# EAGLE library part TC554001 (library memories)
Static RAM 512K x 8 bits Toshiba
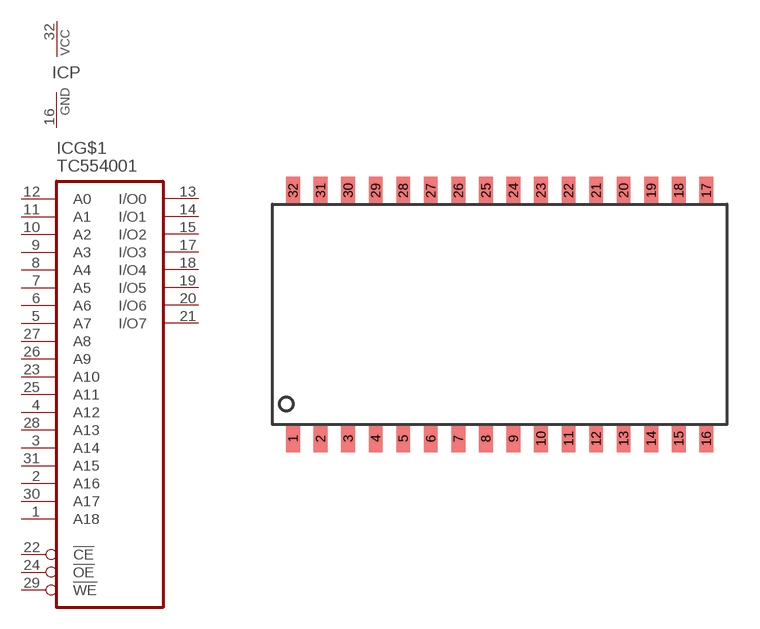
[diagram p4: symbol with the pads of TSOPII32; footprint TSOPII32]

Designator prefix IC; gates G$1=RAM512KX8 P=PWRN

## TC554001T  [TSOPII32]
1  G$1:A18  in
2  G$1:A16  in
3  G$1:A14  in
4  G$1:A12  in
5  G$1:A7  in
6  G$1:A6  in
7  G$1:A5  in
8  G$1:A4  in
9  G$1:A3  in
10  G$1:A2  in
11  G$1:A1  in
12  G$1:A0  in
13  G$1:I/O0  hiz
14  G$1:I/O1  hiz
15  G$1:I/O2  hiz
16  P:GND  pwr
17  G$1:I/O3  hiz
18  G$1:I/O4  hiz
19  G$1:I/O5  hiz
20  G$1:I/O6  hiz
21  G$1:I/O7  hiz
22  G$1:!CE  in
23  G$1:A10  in
24  G$1:!OE  in
25  G$1:A11  in
26  G$1:A9  in
27  G$1:A8  in
28  G$1:A13  in
29  G$1:!WE  in
30  G$1:A17  in
31  G$1:A15  in
32  P:VCC  pwr

## Footprint TSOPII32 (pad centres in mm)
TSOP II32 pins
smd 0.635 x 1.27: 1 -9.525,-5.715; 2 -8.255,-5.715; 3 -6.985,-5.715; 4 -5.715,-5.715; 5 -4.445,-5.715; 6 -3.175,-5.715; 7 -1.905,-5.715; 8 -0.635,-5.715; 9 0.635,-5.715; 10 1.905,-5.715; 11 3.175,-5.715; 12 4.445,-5.715; 13 5.715,-5.715; 14 6.985,-5.715; 15 8.255,-5.715; 16 9.525,-5.715; 17 9.525,5.715; 18 8.255,5.715; 19 6.985,5.715; 20 5.715,5.715; 21 4.445,5.715; 22 3.175,5.715; 23 1.905,5.715; 24 0.635,5.715; 25 -0.635,5.715; 26 -1.905,5.715; 27 -3.175,5.715; 28 -4.445,5.715; 29 -5.715,5.715; 30 -6.985,5.715; 31 -8.255,5.715; 32 -9.525,5.715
